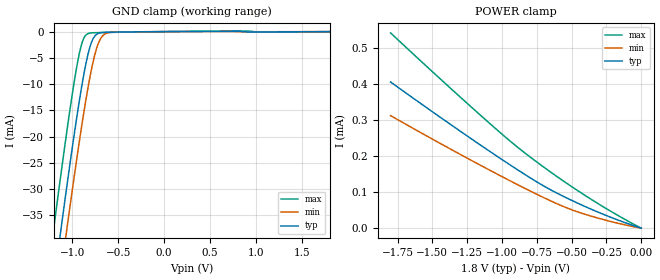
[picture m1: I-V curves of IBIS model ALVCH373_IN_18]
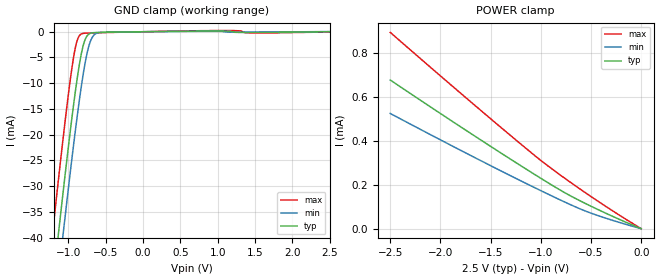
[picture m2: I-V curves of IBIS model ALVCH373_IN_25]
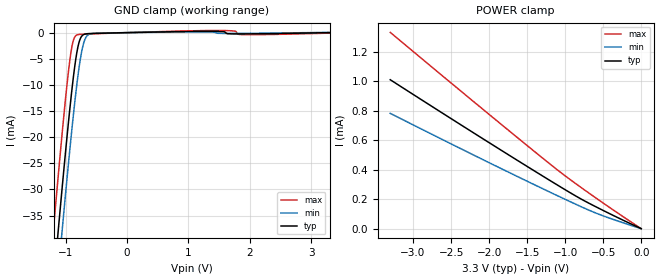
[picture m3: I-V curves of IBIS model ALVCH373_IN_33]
| TEXAS INSTRUMENTS INCORPORATED
| Standard Linear and Logic Group
| IBIS Model of SN74ALVCH373
| OCTAL TRANSPARENT D-TYPE LATCH WITH 3-STATE OUTPUTS
| This file contains package information for the following:
|  TSSOP 20-pin (PW) package as [Component] ALVCH373_PW
|  SOIC 20-pin (DW) package as [Component] ALVCH373_DW
|  TVSOP 20-pin (DGV) package as [Component] ALVCH373_DGV
| This device can be powered at the following Vccs:
|  1.8 volt Vcc
|  2.5 volt Vcc
|  3.3 volt Vcc
| This file provides unique models under the [Model Selector] for each Vcc.
| For operation at a specific Vcc, select the appropriate model after each
| [Model Selector] keyword.
[IBIS Ver]   3.2
[Comment char]  |_char
[File Name]   sn74alvch373.ibs
[File Rev]   1.1 | x_die
[Date]   March 13, 2002
[Source]   Data created from TI-SPICE simulations at TI-SLL.
[Notes]   The following is an IBIS list for the ALVCH373_MH.
   Please contact sllibis@ti.com with questions and
   comments concerning SLL IBIS models.
   Non-monotonic warning due to bus hold circuit.
   Non-monotonic data in pulldown due to feedback circuit in
   output.
   C_comp values are taken at a different test condition than
   the data sheet.
[Disclaimer] Property of Texas Instruments Incorporated.  Unauthorized
   reproduction and/or distribution is strictly prohibited.
   This product is protected under copyright law.
   Created  2002, (C) Copyright  2002, Texas Instruments
   Incorporated, All Rights Reserved
   UNLESS THERE IS A SIGNED, WRITTEN AGREEMENT TO THE
   CONTRARY, TEXAS INSTRUMENTS (TI) IS PROVIDING THE IBIS
   MODELS  AND WITHOUT ANY WARRANTY, EXPRESSED OR
   IMPLIED.  TI assumes no liability for:
   1) the accuracy of the IBIS models provided to your
   company;
   2) the proper functioning of these IBIS Models in your
   design or for any resulting applications; or
   3) infringement of patents, copyrights or intellectual
   property rights resulting from your use of these IBIS
   models.
   TI provides IBIS Models as a service to our customers.
   You and your company shall not distribute, sell or give
   these models to anyone else without prior written
   permission from TI.
   TI reserves the right to make changes to our products or
   to discontinue any semiconductor product or service
   without notice, and advises our customers to obtain the
   latest version of relevant information to verify, before
   placing orders, that the information being relied on is
   current.
   Please be aware that your receipt and use of the IBIS
   information provided shall serve as acceptance of these
   terms and conditions.  If you do not accept these terms,
   you should return or destroy the IBIS models and any
   other accompanying information immediately.
| Component ALVCH373_PW 20-pin TSSOP
[Component]   ALVCH373_PW
[Manufacturer]   Texas Instruments, Inc.
[Package]
|   typ   min   max
R_pkg   4.500e-02   3.600e-02   5.700e-02
L_pkg   2.694e-09   2.290e-09   3.177e-09
C_pkg   1.560e-13   7.600e-14   2.590e-13
[Pin]   signal_name   model_name   R_pin   L_pin   C_pin
1   NOE   ALVCH373_NOE   3.600e-02   3.045e-09   2.590e-13
2   1Q   ALVCH373_OUT   5.100e-02   3.013e-09   1.890e-13
3   1D   ALVCH373_IN   4.400e-02   2.695e-09   1.640e-13
4   2D   ALVCH373_IN   4.700e-02   2.362e-09   7.900e-14
5   2Q   ALVCH373_OUT   4.700e-02   2.333e-09   8.600e-14
6   3Q   ALVCH373_OUT   4.700e-02   2.298e-09   8.500e-14
7   3D   ALVCH373_IN   4.700e-02   2.351e-09   7.900e-14
8   4D   ALVCH373_IN   4.400e-02   2.706e-09   1.650e-13
9   4Q   ALVCH373_OUT   4.900e-02   2.999e-09   1.880e-13
10   GND   GND   3.900e-02   3.039e-09   2.570e-13
11   LE   ALVCH373_LE   3.800e-02   3.044e-09   2.580e-13
12   5Q   ALVCH373_OUT   5.700e-02   3.177e-09   1.990e-13
13   5D   ALVCH373_IN   4.400e-02   2.825e-09   1.730e-13
14   6D   ALVCH373_IN   4.700e-02   2.429e-09   8.300e-14
15   6Q   ALVCH373_OUT   4.900e-02   2.383e-09   9.000e-14
16   7Q   ALVCH373_OUT   4.900e-02   2.347e-09   8.900e-14
17   7D   ALVCH373_IN   4.700e-02   2.290e-09   7.600e-14
18   8D   ALVCH373_IN   4.500e-02   2.613e-09   1.580e-13
19   8Q   ALVCH373_OUT   4.400e-02   2.883e-09   1.810e-13
20   VCC   POWER   3.900e-02   3.044e-09   2.560e-13
| Component ALVCH373_DW 20-pin SOIC
[Component]   ALVCH373_DW
[Manufacturer]   Texas Instruments, Inc.
[Package]
|   typ   min   max
R_pkg   3.800e-02   3.300e-02   4.500e-02
L_pkg   5.012e-09   4.110e-09   6.349e-09
C_pkg   7.170e-13   5.300e-13   8.680e-13
[Pin]   signal_name   model_name   R_pin   L_pin   C_pin
1   NOE   ALVCH373_NOE   4.200e-02   6.336e-09   8.650e-13
2   1Q   ALVCH373_OUT   4.300e-02   5.542e-09   8.670e-13
3   1D   ALVCH373_IN   3.400e-02   4.714e-09   7.320e-13
4   2D   ALVCH373_IN   3.400e-02   4.377e-09   5.910e-13
5   2Q   ALVCH373_OUT   3.600e-02   4.130e-09   5.330e-13
6   3Q   ALVCH373_OUT   3.500e-02   4.111e-09   5.300e-13
7   3D   ALVCH373_IN   3.400e-02   4.284e-09   5.830e-13
8   4D   ALVCH373_IN   3.400e-02   4.634e-09   7.260e-13
9   4Q   ALVCH373_OUT   4.000e-02   5.518e-09   8.650e-13
10   GND   GND   4.300e-02   6.349e-09   8.660e-13
11   LE   ALVCH373_LE   4.100e-02   6.281e-09   8.610e-13
12   5Q   ALVCH373_OUT   4.500e-02   5.561e-09   8.680e-13
13   5D   ALVCH373_IN   3.300e-02   4.778e-09   7.420e-13
14   6D   ALVCH373_IN   3.500e-02   4.414e-09   5.960e-13
15   6Q   ALVCH373_OUT   3.500e-02   4.110e-09   5.330e-13
16   7Q   ALVCH373_OUT   3.600e-02   4.130e-09   5.330e-13
17   7D   ALVCH373_IN   3.400e-02   4.377e-09   5.910e-13
18   8D   ALVCH373_IN   3.400e-02   4.714e-09   7.310e-13
19   8Q   ALVCH373_OUT   4.300e-02   5.569e-09   8.680e-13
20   VCC   POWER   4.200e-02   6.308e-09   8.640e-13
| Component ALVCH373_DGV 20-pin TVSOP
[Component]   ALVCH373_DGV
[Manufacturer]   Texas Instruments, Inc.
[Package]
|   typ   min   max
R_pkg   4.400e-02   3.800e-02   4.800e-02
L_pkg   2.561e-09   2.236e-09   2.961e-09
C_pkg   3.420e-13   2.640e-13   4.460e-13
[Pin]   signal_name   model_name   R_pin   L_pin   C_pin
1   NOE   ALVCH373_NOE   4.400e-02   2.935e-09   4.170e-13
2   1Q   ALVCH373_OUT   4.200e-02   2.869e-09   4.460e-13
3   1D   ALVCH373_IN   4.300e-02   2.399e-09   3.160e-13
4   2D   ALVCH373_IN   4.400e-02   2.236e-09   2.650e-13
5   2Q   ALVCH373_OUT   4.600e-02   2.278e-09   2.640e-13
6   3Q   ALVCH373_OUT   4.500e-02   2.274e-09   2.640e-13
7   3D   ALVCH373_IN   4.400e-02   2.285e-09   2.690e-13
8   4D   ALVCH373_IN   4.300e-02   2.452e-09   3.200e-13
9   4Q   ALVCH373_OUT   4.400e-02   2.900e-09   4.460e-13
10   GND   GND   4.400e-02   2.961e-09   4.180e-13
11   LE   ALVCH373_LE   4.500e-02   2.954e-09   4.180e-13
12   5Q   ALVCH373_OUT   4.200e-02   2.847e-09   4.430e-13
13   5D   ALVCH373_IN   4.500e-02   2.453e-09   3.190e-13
14   6D   ALVCH373_IN   4.500e-02   2.297e-09   2.690e-13
15   6Q   ALVCH373_OUT   4.800e-02   2.334e-09   2.680e-13
16   7Q   ALVCH373_OUT   4.800e-02   2.335e-09   2.670e-13
17   7D   ALVCH373_IN   4.600e-02   2.299e-09   2.680e-13
18   8D   ALVCH373_IN   4.600e-02   2.457e-09   3.200e-13
19   8Q   ALVCH373_OUT   4.300e-02   2.848e-09   4.410e-13
20   VCC   POWER   3.800e-02   2.812e-09   4.080e-13
| Model ALVCH373_IN
[Model Selector]   ALVCH373_IN
ALVCH373_IN_18   1.8 volt Vcc
ALVCH373_IN_25   2.5 volt Vcc
ALVCH373_IN_33   3.3 volt Vcc
| Model ALVCH373_LE
[Model Selector]   ALVCH373_LE
ALVCH373_LE_18   1.8 volt Vcc
ALVCH373_LE_25   2.5 volt Vcc
ALVCH373_LE_33   3.3 volt Vcc
| Model ALVCH373_NOE
[Model Selector]   ALVCH373_NOE
ALVCH373_NOE_18   1.8 volt Vcc
ALVCH373_NOE_25   2.5 volt Vcc
ALVCH373_NOE_33   3.3 volt Vcc
| Model ALVCH373_OUT
[Model Selector]   ALVCH373_OUT
ALVCH373_OUT_18   1.8 volt Vcc
ALVCH373_OUT_25   2.5 volt Vcc
ALVCH373_OUT_33   3.3 volt Vcc
| Models and submodels in the file (12): ALVCH373_IN_18 (Input), ALVCH373_IN_25 (Input), ALVCH373_IN_33 (Input), ALVCH373_LE_18 (Input), ALVCH373_LE_25 (Input), ALVCH373_LE_33 (Input), ALVCH373_NOE_18 (Input), ALVCH373_NOE_25 (Input), ALVCH373_NOE_33 (Input), ALVCH373_OUT_18 (3-state), ALVCH373_OUT_25 (3-state), ALVCH373_OUT_33 (3-state)
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[Model]   ALVCH373_IN_18
Model_type  Input
Vinl=0.5775
Vinh=1.2675
| variable   typ   min   max
C_comp   4.45pF   3.77pF   5.53pF
[Temperature Range]   40   100   -40
| Ambient temperature   25   85   -40
[Voltage range]   1.8   1.65   1.95
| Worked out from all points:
|   GND clamp passes 1 mA (typ) near -0.76 V on its own axis
[GND Clamp]
| ALVCH373_IN_18
|   Voltage   I(typ)   I(min)   I(max)
-1.8V     -130.2mA   -138.1mA   -120.2mA
-1.205V   -48.52mA   -56.73mA   -38mA
-1.125V   -38mA      -46.21mA   -27.47mA
-1.06V    -29.66mA   -37.84mA   -19.2mA
-930mV    -14.03mA   -21.82mA   -4.811mA
-885mV    -9.27mA    -16.66mA   -1.737mA
-840mV    -5.206mA   -11.86mA   -501.3uA
-785mV    -1.818mA   -6.734mA   -237.2uA
-725mV    -419.1uA   -2.685mA   -196.4uA
-675mV    -173.7uA   -933uA     -178.7uA
-605mV    -109.7uA   -195.8uA   -156.2uA
1.8V      4.859pA    12.08uA    -28.71uA
[POWER Clamp]
| ALVCH373_IN_18
|   Voltage   I(typ)   I(min)   I(max)
-1.8V     406.2uA    312.7uA    542.6uA
-1.19V    240.4uA    182.1uA    326.1uA
-980mV    185.6uA    139.2uA    254.6uA
-845mV    151.6uA    112.5uA    211.8uA
-665mV    109.6uA    78.5uA     159.9uA
-465mV    71.04uA    46.41uA    106.5uA
-235mV    32.73uA    20.13uA    50.68uA
-16.28fV  4.859pA    7.93pA     4.983pA
[Model]   ALVCH373_IN_25
Model_type  Input
Vinl=0.7
Vinh=1.7
| variable   typ   min   max
C_comp   4.43pF   3.59pF   5.38pF
[Temperature Range]   40   100   -40
| Ambient temperature   25   85   -40
[Voltage range]   2.5   2.3   2.7
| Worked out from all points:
|   GND clamp passes 1 mA (typ) near -0.76 V on its own axis
[GND Clamp]
| ALVCH373_IN_25
|   Voltage   I(typ)   I(min)   I(max)
-2.5V     -228.8mA   -236.3mA   -219.5mA
-1.23V    -51.91mA   -60.1mA    -41.43mA
-1.2V     -47.92mA   -56.11mA   -37.42mA
-1.13V    -38.71mA   -46.91mA   -28.19mA
-1.07V    -30.98mA   -39.15mA   -20.52mA
-925mV    -13.52mA   -21.27mA   -4.453mA
-880mV    -8.824mA   -16.14mA   -1.576mA
-830mV    -4.484mA   -10.89mA   -463.8uA
-775mV    -1.478mA   -5.958mA   -283.8uA
-720mV    -414.1uA   -2.472mA   -249.6uA
-610mV    -146.8uA   -241.8uA   -206.5uA
2.5V      6.656pA    26.03uA    -53.38uA
[POWER Clamp]
| ALVCH373_IN_25
|   Voltage   I(typ)   I(min)   I(max)
-2.5V     677.9uA    525.3uA    895.1uA
-1.605V   406.5uA    311.8uA    542uA
-985mV    225.4uA    170.1uA    305.9uA
-745mV    159.8uA    117.9uA    224.5uA
-525mV    107.9uA    74.99uA    154.2uA
-280mV    55.17uA    37.23uA    79.94uA
-31.15fV  6.656pA    9.568pA    6.889pA
[Model]   ALVCH373_IN_33
Model_type  Input
Vinl=0.8
Vinh=2.0
| variable   typ   min   max
C_comp   4.37pF   3.43pF   5.36pF
[Temperature Range]   40   100   -40
| Ambient temperature   25   85   -40
[Voltage range]   3.3   3   3.6
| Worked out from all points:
|   GND clamp passes 1 mA (typ) near -0.76 V on its own axis
|   POWER clamp passes 1 mA (typ) near -3.27 V on its own axis
[GND Clamp]
| ALVCH373_IN_33
|   Voltage   I(typ)   I(min)   I(max)
-3.3V     -342.6mA   -349.7mA   -333.8mA
-1.215V   -49.97mA   -58.14mA   -39.5mA
-1.185V   -45.99mA   -54.17mA   -35.5mA
-1.125V   -38.11mA   -46.3mA    -27.62mA
-1.065V   -30.4mA    -38.55mA   -19.97mA
-925mV    -13.57mA   -21.3mA    -4.518mA
-875mV    -8.384mA   -15.63mA   -1.438mA
-820mV    -3.821mA   -9.942mA   -457.1uA
-770mV    -1.353mA   -5.601mA   -335.7uA
-715mV    -413.1uA   -2.272mA   -301uA
-585mV    -169.2uA   -185.2uA   -242.5uA
3.3V      8.672pA    50.51uA    -98.23uA
[POWER Clamp]
| ALVCH373_IN_33
|   Voltage   I(typ)   I(min)   I(max)
-3.3V     1.009mA    781uA      1.329mA
-1.985V   577.7uA    443.1uA    767.6uA
-1.09V    291.8uA    220.4uA    393.1uA
-810mV    206.4uA    153.4uA    286uA
-575mV    142.7uA    101.3uA    200.3uA
-48.03fV  8.672pA    11.32pA    9.138pA
